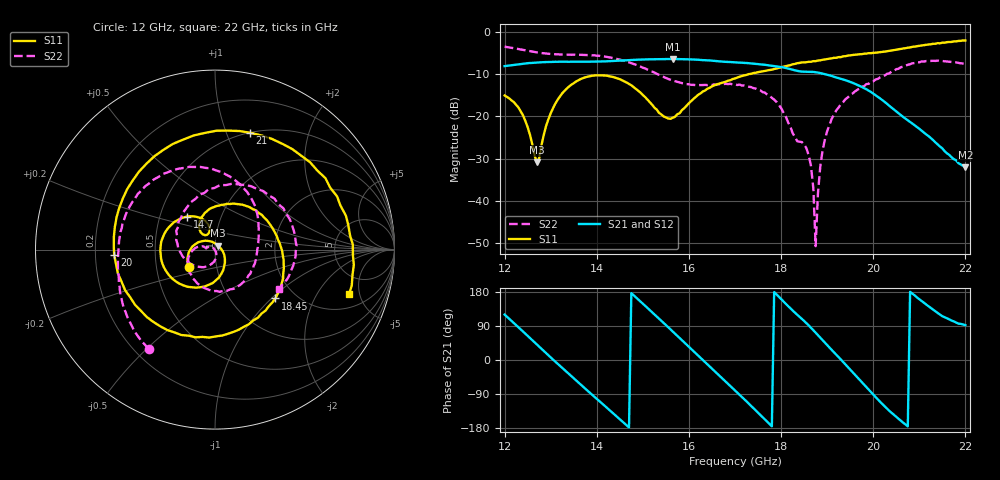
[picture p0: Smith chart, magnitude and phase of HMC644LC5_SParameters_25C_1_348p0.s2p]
!Analog Devices Inc..
!GaAs MMIC 5-BIT DIGITAL PHASE SHIFTER, 15 -8.5 GHz
!Filename: HMC644LC5_sparm_25C_1_0.s2p
!  :25C = 25degC
!  :_1_ = Sn1
!  :_348p0  = 348.75deg
!Device type:
!2 Port Calibration to sma connectors
!Phase Shifter:  0.000
!	50 Ohm System, Control Voltage = 0/-3V
!Freq	S11	S11	S21	S21	S12	S12	S22	S22
! GHz	Mag dB	Degrees	Mag dB	Degrees	Mag dB	Degrees	Mag dB	Degrees
# GHZ S DB R 50.0
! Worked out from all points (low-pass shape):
!   201 points, 12 GHz to 22 GHz, reference 50 ohm
!   highest |S21| = -6.45 dB at 15.65 GHz (marker M1); lowest = -32.1 dB at 22 GHz (marker M2)
!   |S21| within 3 dB of the highest: start of sweep to 18.48 GHz
!   lowest |S11| = -30.9 dB at 12.7 GHz (marker M3), VSWR 1.06, Z = 51.8 + j2.3 ohm
!   |S11| at or under -10 dB: start of sweep to 17.32 GHz
!   |S22| runs from -50.7 to -3.5 dB; largest |S21 - S12| = 0.0025
!   S11 on the Smith chart (normalised r, x): 12 GHz: 0.73, -0.15; 14.7 GHz: 0.69, +0.27; 18.45 GHz: 1.58, -1.06; 20 GHz: 0.28, -0.02; 21 GHz: 0.50, +1.22; 22 GHz: 3.03, -3.95
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12  -15.09 -146.9  -8.14 119.9  -8.14 119.9  -3.52 -123.7
12.4  -19.80 156.4  -7.57 75.1  -7.57 75.2  -4.32 -144.9
12.7  -30.90 51.1  -7.27 40.8  -7.28 40.9  -4.89 -159.1
13.1  -17.03 -76.0  -7.11 -4.3  -7.12 -4.3  -5.34 -176.6
13.7  -11.00 -141.4  -7.10 -70.3  -7.09 -70.3  -5.47 153.0
14.7  -12.36 130.2  -6.72 -178.0  -6.72 -177.9  -7.25 85.7
15.35  -19.19 105.5  -6.47 109.2  -6.46 109.2  -10.20 40.6
15.65  -20.34 123.0  -6.45 75.0  -6.45 75.1  -11.56 23.1
16.3  -14.15 112.3  -6.72 0.1  -6.69 0.2  -12.62 -16.2
17  -11.06 65.6  -7.26 -80.0  -7.24 -80.0  -12.43 -73.9
17.75  -9.06 12.2  -7.99 -168.9  -7.96 -168.9  -15.16 -150.6
18.45  -7.28 -39.0  -9.44 108.6  -9.42 108.6  -26.11 173.1
18.7  -6.96 -57.7  -9.51 78.7  -9.51 78.6  -37.09 139.2
18.75  -6.97 -61.6  -9.59 72.1  -9.56 72.1  -50.73 163.9
18.85  -6.77 -69.1  -9.78 58.9  -9.78 59.0  -31.97 -73.6
19  -6.47 -81.4  -10.18 39.3  -10.16 39.2  -23.51 -93.8
19.5  -5.60 -125.4  -11.87 -25.3  -11.87 -25.1  -14.98 -163.8
20  -5.00 -176.9  -14.63 -91.3  -14.58 -91.2  -11.75 137.3
20.35  -4.52 145.3  -17.54 -134.4  -17.52 -134.0  -9.84 100.3
21  -3.35 73.3  -22.96 160.3  -22.91 160.2  -7.25 35.9
21.5  -2.59 23.5  -27.60 115.5  -27.70 116.3  -6.93 -4.7
22  -2.08 -18.4  -32.08 91.8  -32.12 92.1  -7.55 -31.5
